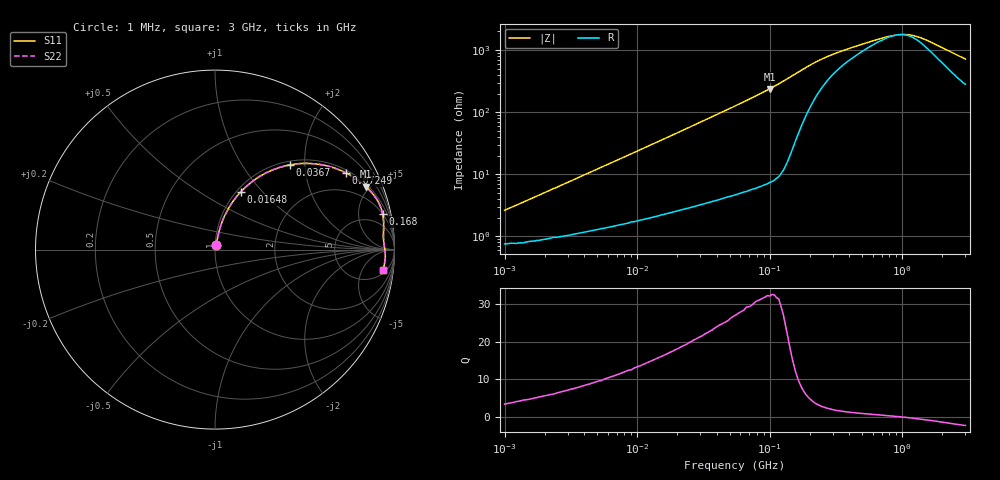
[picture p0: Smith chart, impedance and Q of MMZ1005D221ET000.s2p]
! S-parameter Generated by TDK Corporation
! Copyright(C) 2016 TDK Corporation.
! All Rights Reserved.
! TDK P/N: MMZ1005D221ET000 (Chip Beads)
! Property: |Z|=220¶ at 100MHz
! Size(LxWxT): 1x0.5x0.5mm, 0.039x0.02x0.02inches
! Model Type: s2p (Touchstone File Format Version 1.0)
! Frequency: DC=Yes Start=1MHz Stop=3000MHz 202points Log-sweep
! Note: This model was converted from impedance.
! Model Generated on May. 16, 2016
! Hash(MD5):
! Port Assignments:
!  1 ---@@@--- 2
! Applicable Conditions:
!  Temperature = 25 degC
!  DC Bias Current = 0 A
!  Small Signal Operation
! Terms and conditions regarding TDK Simulation Models
! (1)This simulation model is being provided solely for informational purposes. Please refer to the specifications of the products in terms of detailed characteristics of such products.
! (2)In no event shall TDK Corporation of any of its subsidiaries be liable for any loss or damage arising, directly or indirectly,
!  From any information contained in this simulation model, including, but not limited to loss or damages arising from any inaccuracies, omissions or errors in connection with such information.
! (3)Any and all copyrights on this simulation model are owned by TDK Corporation.
!  Duplication or redistribution of this simulation model without prior written permission from TDK Corporation is prohibited.
! (4)This simulation model is subject to any modification or change without any prior notice.
! (5)Neither TDK Corporation nor any of its subsidiaries shall make any warranty, express or implied,
!  Including but not limited to the correctness, implied warranties of merchantability and fitness for a particular purpose with respect to this simulation models.
! (6)The use of this simulation model shall be deemed to have consented to the terms and conditions hereof.
# MHz S MA R 50
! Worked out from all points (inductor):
!   201 points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, 1 MHz to 3 GHz, reference 50 ohm
!   read as one part in series: L = 401 nH near 1.041 MHz
!   highest Q = 32.3 at 99.85 MHz (marker M1), where L = 378 nH
!   self-resonance near 941 MHz
!   S11 on the Smith chart (normalised r, x): 1 MHz: 1.02, +0.05; 16.48 MHz: 1.05, +0.77; 36.7 MHz: 1.07, +1.68; 72.49 MHz: 1.11, +3.36; 168 MHz: 2.01, +9.07; 3 GHz: 7, -13
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1  0.02624 71.9  0.9922 -1.4  0.9922 -1.4  0.02624 71.9
2.055611  0.05141 77.1  0.9897 -2.9  0.9897 -2.9  0.05141 77.1
3.900413  0.09411 77.7  0.9842 -5.4  0.9842 -5.4  0.09411 77.7
8.345207  0.1915 74.3  0.966 -11.0  0.966 -11.0  0.1915 74.3
14.61624  0.317 67.9  0.9286 -18.4  0.9286 -18.4  0.317 67.9
16.48134  0.3513 66.0  0.9154 -20.5  0.9154 -20.5  0.3513 66.0
24.59509  0.4832 58.2  0.8514 -28.9  0.8514 -28.9  0.4832 58.2
36.70325  0.6309 48.4  0.7491 -39.1  0.7491 -39.1  0.6309 48.4
54.77226  0.7692 37.6  0.6111 -50.2  0.6111 -50.2  0.7692 37.6
72.48696  0.8467 30.3  0.5043 -57.8  0.5043 -57.8  0.8467 30.3
99.84923  0.9115 22.6  0.3839 -65.7  0.3839 -65.7  0.9115 22.6
132.1429  0.9471 16.5  0.284 -71.1  0.284 -71.1  0.9471 16.5
168.0187  0.955 12.0  0.2093 -71.6  0.2093 -71.6  0.955 12.0
213.6344  0.9508 8.6  0.1549 -67.2  0.1549 -67.2  0.9508 8.6
271.6345  0.9449 6.3  0.1203 -59.6  0.1203 -59.6  0.9449 6.3
359.4878  0.9412 4.4  0.0953 -49.7  0.0953 -49.7  0.9412 4.4
655.3423  0.943 1.6  0.06294 -24.4  0.06294 -24.4  0.943 1.6
800.5644  0.9448 0.7  0.05658 -12.2  0.05658 -12.2  0.9448 0.7
1017.911  0.9473 -0.4  0.05303 6.4  0.05303 6.4  0.9473 -0.4
1294.266  0.9491 -1.6  0.05734 26.7  0.05734 26.7  0.9491 -1.6
1581.072  0.9496 -2.7  0.06773 40.6  0.06773 40.6  0.9496 -2.7
3000  0.9415 -6.9  0.1309 60.0  0.1309 60.0  0.9415 -6.9
